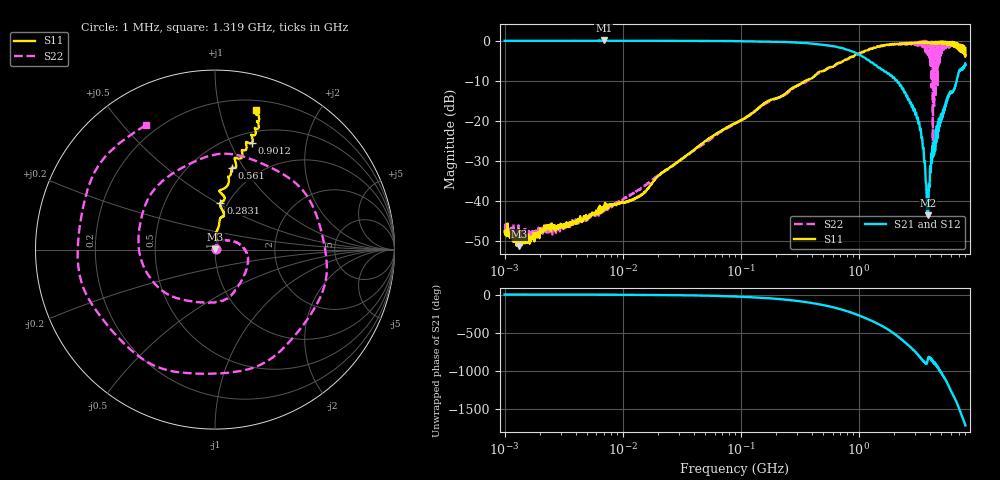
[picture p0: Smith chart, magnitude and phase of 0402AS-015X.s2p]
!s-Parameter Generated by FASTRON Sdn. Bhd.
!FASTRON P/N : 0402AS-015X
!Keysight Technologies: E5071C_MY46733604_B.14.02
!Date: Mon Dec 01 10:31:17 2025
!Version  :Rev00  Mon Dec 01 10:31:17 2025
!Data & Calibration Information:
!Freq  S11:SOLT2(ON)  S21:SOLT2(ON)  S12:SOLT2(ON)  S22:SOLT2(ON)
!PortZ  Port1:50+j0  Port2:50+j0
!When reading reference impedance value at option line is always used.
! Remarks : This data is being provided solely for informational purposes.
# Hz S dB R 50
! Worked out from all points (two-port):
!   1601 points, 1 MHz to 8 GHz, reference 50 ohm
!   highest |S21| = 0.04 dB at 6.912 MHz (marker M1); lowest = -43.6 dB at 3.852 GHz (marker M2)
!   |S21| within 3 dB of the highest: start of sweep to 927.1 MHz
!   lowest |S11| = -51.3 dB at 1.323 MHz (marker M3), VSWR 1.01, Z = 50.2 + j0.126 ohm
!   |S11| at or under -10 dB: start of sweep to 353.6 MHz
!   |S22| runs from -49.7 to 0.0 dB; largest |S21 - S12| = 0.015
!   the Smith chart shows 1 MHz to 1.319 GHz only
!   S11 on the Smith chart (normalised r, x): 1 MHz: 1.01, +0.00; 283.1 MHz: 0.92, +0.52; 561 MHz: 0.76, +0.88; 901.2 MHz: 0.61, +1.21; 1.319 GHz: 0.29, +1.30
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1000000  -47.60 26.9  -0.05 -0.2  -0.03 -0.3  -46.60 22.3
1323440  -51.30 27.4  -0.04 -0.4  -0.04 -0.4  -47.60 11.1
4479405  -44.60 50.1  -0.04 -1.4  -0.03 -1.4  -44.70 54.0
6911657  -41.40 41.7  0.04 -2.2  0.02 -2.2  -41.30 49.1
2.00676e7  -33.70 68.5  -0.05 -5.8  -0.05 -5.8  -33.60 71.4
8.994653e7  -20.60 85.6  -0.13 -25.5  -0.12 -25.5  -20.70 33.3
2.831256e8  -11.60 83.4  -0.46 -79.1  -0.45 -79.1  -11.70 -65.8
4.006501e8  -9.40 82.9  -0.73 -111.0  -0.72 -111.0  -9.27 -128.0
5.610091e8  -6.65 78.5  -1.27 -155.0  -1.26 -155.0  -6.83 151.0
9.011973e8  -4.00 70.9  -2.84 114.0  -2.83 114.0  -3.82 -24.3
1.069649e9  -2.96 71.3  -3.96 69.6  -3.96 69.5  -2.80 -113.0
1.318613e9  -1.85 73.6  -5.59 7.9  -5.59 7.7  -2.01 119.0
1.558366e9  -1.35 77.2  -7.24 -48.4  -7.25 -48.5  -1.24 3.2
1.7949e9  -1.03 82.0  -8.19 -104.0  -8.20 -104.0  -1.17 -113.0
2.103821e9  -0.78 87.8  -9.98 179.0  -9.98 179.0  -1.00 88.4
2.457552e9  -0.86 91.9  -12.90 96.8  -12.80 96.7  -0.78 -80.4
2.648292e9  -0.83 96.5  -14.70 54.1  -14.60 54.0  -0.65 -171.0
2.839031e9  -0.74 101.0  -16.40 11.8  -16.40 11.6  -0.52 98.4
3.162936e9  -0.52 109.0  -19.30 -68.7  -19.30 -69.0  -1.31 -74.8
3.548043e9  -0.39 118.0  -27.60 -161.0  -27.60 -162.0  -2.18 79.0
3.852076e9  -0.46 123.0  -43.60 -131.0  -43.60 -131.0  -3.58 -82.7
8e9  -1.91 -109.0  -6.08 85.1  -6.10 84.7  -3.22 117.0
